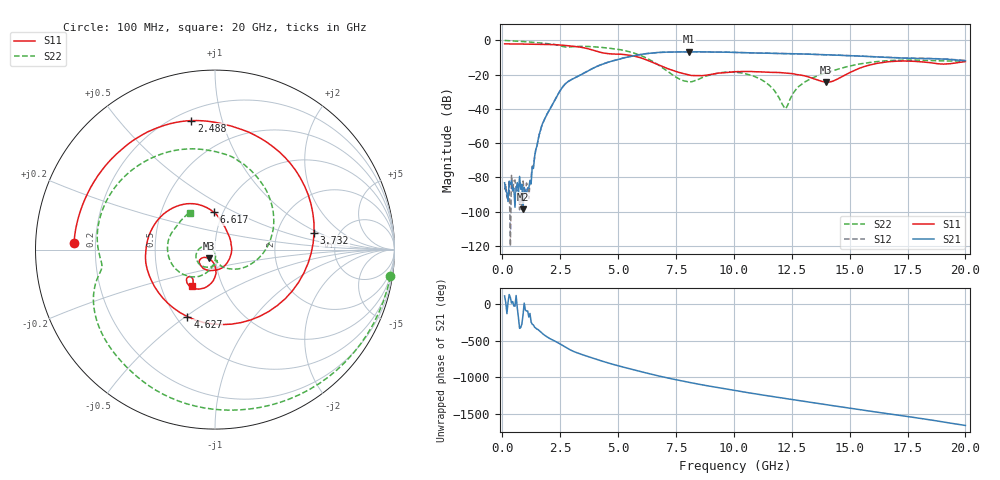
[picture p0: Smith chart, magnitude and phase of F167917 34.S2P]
!  2-Port S-parameters saved by WinCal
! VAR MeasName=S-Parameters (CALIBRATED_DATA) read from VNA (N5242A)
! VAR MeasDate=2016-11-22 9:01:26
! VAR NAME=F167917 34
! VAR FILENAME=F167917 34.S2P
! VAR DATE=2016-11-22 9:01:26
! VAR PHYS_PORTS=1,2
# Hz S DB R 50
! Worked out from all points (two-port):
!   401 points, 100 MHz to 20 GHz, reference 50 ohm
!   highest |S21| = -6.66 dB at 8.06 GHz (marker M1); lowest = -98.7 dB at 896 MHz (marker M2)
!   |S21| within 3 dB of the highest: 5.457 GHz to 16.14 GHz (10.68 GHz wide, 98.9 % of centre)
!   lowest |S11| = -24.5 dB at 13.98 GHz (marker M3), VSWR 1.13, Z = 46.5 - j4.6 ohm
!   |S11| at or under -10 dB: 5.918 GHz to end of sweep
!   |S22| runs from -39.8 to -0.1 dB; largest |S21 - S12| = 0.0053
!   S11 on the Smith chart (normalised r, x): 100 MHz: 0.12, +0.02; 2.488 GHz: 0.26, +0.80; 3.732 GHz: 3.28, +0.88; 4.627 GHz: 0.57, -0.51; 6.617 GHz: 0.90, +0.39; 20 GHz: 0.72, -0.31
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1e8  -2.09 177.3  -83.12 116.1  -87.14 52.8  -0.10 -8.7
8.96e8  -2.21 156.1  -98.68 -144.0  -82.11 -11.8  -0.72 -70.4
1.24425e9  -2.26 146.2  -83.81 117.7  -80.15 131.0  -1.07 -94.0
1.74175e9  -2.36 130.7  -48.46 -42.0  -48.45 -43.4  -1.68 -124.3
2.488e9  -2.73 100.3  -29.59 178.4  -29.60 178.2  -3.17 -163.9
3.43325e9  -4.14 40.0  -19.83 32.6  -19.85 32.6  -3.54 164.3
3.73175e9  -5.04 9.5  -17.62 0.9  -17.64 1.1  -3.62 150.7
4.22925e9  -6.98 -56.1  -14.43 -50.4  -14.40 -50.3  -4.08 127.4
4.62725e9  -7.88 -112.3  -12.57 -88.8  -12.51 -88.9  -4.63 107.7
5.72175e9  -9.31 141.8  -8.91 178.4  -8.91 178.0  -7.60 42.9
6.61725e9  -13.60 92.1  -7.22 108.2  -7.27 108.1  -13.33 -22.0
6.7665e9  -14.46 86.0  -7.08 97.1  -7.12 97.0  -14.63 -33.3
8.06e9  -20.17 25.5  -6.66 10.8  -6.67 10.8  -24.46 -82.3
1.005e10  -18.29 -104.9  -7.06 -102.4  -7.06 -102.3  -18.68 -150.7
1.13435e10  -18.56 -133.5  -7.52 -168.2  -7.50 -168.1  -24.25 163.0
1.218925e10  -19.12 -142.3  -7.77 150.6  -7.75 150.4  -39.55 -155.5
1.338325e10  -22.11 -145.8  -8.18 92.6  -8.17 92.7  -22.08 -94.8
1.398025e10  -24.49 -124.3  -8.47 64.5  -8.44 64.4  -18.95 -103.5
1.527375e10  -17.13 -88.4  -9.11 3.5  -9.07 3.4  -14.21 -128.6
1.67165e10  -12.47 -112.5  -10.01 -63.1  -9.99 -63.0  -11.86 -163.7
1.865675e10  -13.39 -134.5  -10.74 -153.2  -10.70 -153.4  -11.95 151.5
2e10  -12.40 -122.3  -11.87 138.9  -11.77 138.7  -12.12 124.5
